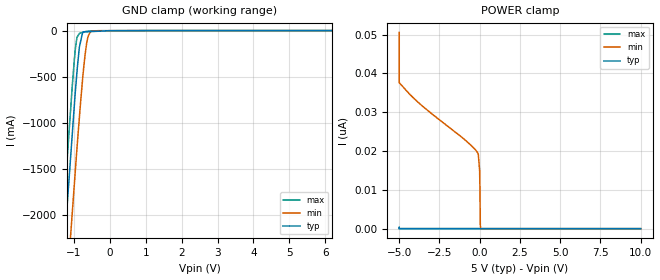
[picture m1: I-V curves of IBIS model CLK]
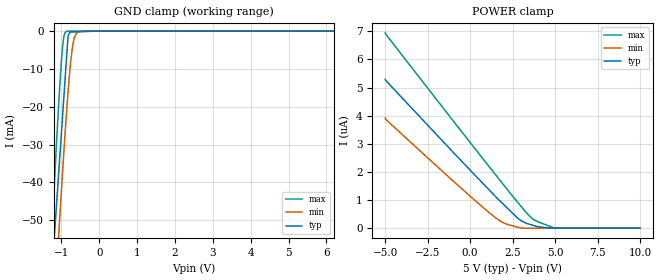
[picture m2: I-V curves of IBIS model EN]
|Texas Instruments Incorporated
| SN6507 Low-Emissions, 36-V Push-Pull Transformer Driver
| Marketing Part # : SN6507
| Package-type: HVSSOP
| #pins/pkg drawing : 10-pin DGQ
[IBIS Ver] 4.1
[File name] sn6507.ibs
[File Rev] 1.0
[Date] 06/27/2022
[Source]
| Texas Instruments Incorporated.
| 12500 TI Blvd
| Dallas, TX -75243
[Notes] Revision History:
| Rev 1.0: 06/27/2022
| - Initial version of the model
| - Model generated from simulations in TISPICE/SPECTRE
| - C_comp although listed in numerical order of value are
| obtained from varying PVT conditions. For PVT conditions for
| each specific value refer the buffer description under
| respective [Model]. IBIS model user is responsible for using
| appropriate C_comp to simulate for Signal Integrity.
| - Warnings regarding combined Non-monotonicity of various models have been
| reviewed and considered minor and can be ignored.
[Disclaimer]
| This model is designed as an aid for customers of Texas Instruments.
| TI and its licensors and suppliers make no warranties, either expressed
| or implied, with respect to this model, including the warranties of
| merchantability or fitness for a particular purpose. The model is
| provided solely on an "as is" basis. The entire risk as to its quality
| and performance is with the customer.
| This model is subject to change without notice. Texas Instruments
| Incorporated is not responsible for updating this model.
[Copyright]
(C) Copyright 2022 Texas Instruments Incorporated. All rights reserved.
| Component1 TCA7408ZSZR (per package)
[Component] SN6507
[Manufacturer] Texas Instruments Incorporated
[Package] |HVSSOP (DGQ) 10-pin
| variable typ min max
R_pkg 0.05 0.04 0.06
L_pkg 1.0nH 0.8nH 1.2nH
C_pkg 0.2pF 0.16pF 0.24pF
| pin number (pin name) mapping to model name
[Pin] signal_name model_name R_pin   L_pin   C_pin
1 SW1 NC NA NA NA
2  GND  GND NA NA NA
3  VCC  POWER NA NA NA
4  EN_UVLO  EN NA NA NA
5  DC  NC NA NA NA
6  SR  NC NA NA NA
7  CLK  CLK NA NA NA
8  SS_ILIM  NC NA NA NA
9  GND  GND NA NA NA
10  SW2  NC NA NA NA
11  PowerPAD  GND NA NA NA
| Models and submodels in the file (2): CLK (Input), EN (Input)
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| Model CLK
[Model]   CLK
Model_type   Input
Vinl = 1.0
Vinh = 1.8
|   typ   min   max
C_comp   5pF   4pF   6pF
[Voltage Range]   5   4   5.5
[Temperature Range]   27   150   -55
[Power Clamp Reference]   5   4   5.5
[GND Clamp Reference]   0   0   0
[GND Clamp]
|   Voltage   I(typ)   I(min)   I(max)
-5V       -18.79A    -18.33A    -19.37A
-1.355V   -2.848A    -3.677A    -2.375A
-1.207V   -1.992A    -2.851A    -1.503A
-1.144V   -1.647A    -2.496A    -1.139A
-1.044V   -1.107A    -1.961A    -585.8mA
-966.8mV  -688.8mA   -1.547A    -221.3mA
-916.9mV  -453.2mA   -1.283A    -74.76mA
-842.5mV  -168mA     -912.1mA   -29.99mA
-762mV    -25.02mA   -539.9mA   -20.43mA
-645.3mV  -13.19mA   -134.7mA   -9.118mA
-497.4mV  -10.39mA   -5.678mA   -2.358mA
10V       0A         0A         0A
[POWER Clamp]
|   Voltage   I(typ)   I(min)   I(max)
-5V       373.1pA    50.56nA    204pA
-5V       0A         37.71nA    0A
-5V       0A         37.62nA    0A
-3.627V   0A         31.82nA    0A
-929.8mV  0A         22.92nA    0A
-333.9mV  0A         20.62nA    0A
-87.74mV  0A         19.23nA    0A
-4.247mV  0A         15.11nA    0A
12.55mV   0A         11.45nA    0A
39.77mV   0A         883.4pA    0A
69.47mV   0A         0A         0A
10V       0A         0A         0A
| Model EN
[Model]   EN
Model_type   Input
Vinl = 1.25
Vinh = 1.6
|   typ   min   max
C_comp   5pF   4pF   6pF
[Voltage Range]   5   4   5.5
[Temperature Range]   27   150   -55
[Power Clamp Reference]   5   4   5.5
[GND Clamp Reference]   0   0   0
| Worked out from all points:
|   GND clamp passes 1 mA (typ) near -0.81 V on its own axis
[GND Clamp]
|   Voltage   I(typ)   I(min)   I(max)
-5V       -2.403A    -1.858A    -2.833A
-2.28V    -276.7mA   -280.5mA   -281.1mA
-1.205V   -57.02mA   -77.55mA   -44.52mA
-1.195V   -55.51mA   -75.62mA   -42.26mA
-1.154V   -49.56mA   -67.95mA   -34.35mA
-1.072V   -37.53mA   -54.12mA   -19.26mA
-968.4mV  -22.36mA   -37.29mA   -4.131mA
-873.5mV  -8.462mA   -22.86mA   -111.6uA
-826.1mV  -1.513mA   -16.46mA   -13.03uA
-708.5mV  -224.9uA   -4.244mA   -8.411uA
-572.2mV  -182uA     -253.5uA   -3.064uA
10V       0A         0A         0A
[POWER Clamp]
|   Voltage   I(typ)   I(min)   I(max)
-5V       5.295uA    3.911uA    6.944uA
-4.915V   5.217uA    3.84uA     6.855uA
-1.154V   2.798uA    1.761uA    3.936uA
221mV     1.925uA    1.018uA    2.876uA
1.574V    1.075uA    336.1nA    1.842uA
2.074V    781.1nA    160.9nA    1.463uA
2.809V    350.3nA    32.16nA    914.2nA
3.292V    177.2nA    0A         566nA
3.65V     110.4nA    0A         345.1nA
4.542V    11.22nA    0A         96.95nA
5.176V    0A         0A         0A
10V       0A         0A         0A
